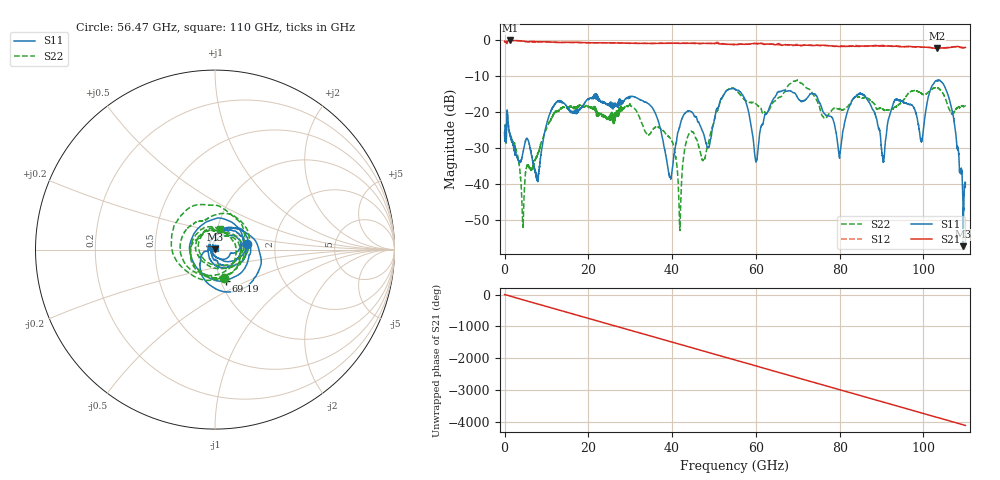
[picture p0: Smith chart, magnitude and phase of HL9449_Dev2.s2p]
! 5/9/2022 12:37:12 PM
! C:\USERS\VECTORSTARUSER\DESKTOP\JASON\HL9449-11\HL9449-11-NE04.S2P
! CHANNEL.1
! TR.MEASUREMENT
! CORRECTED.DATA
# GHZ S RI R 50.0
! FREQ.GHZ  S11RE  S11IM  S21RE  S21IM  S12RE  S12IM  S22RE  S22IM
!; PortSelection: Port_12
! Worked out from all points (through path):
!   5000 points, 22 MHz to 110 GHz, reference 50 ohm
!   highest |S21| = -0.24 dB at 1.386 GHz (marker M1); lowest = -2.4 dB at 103.2 GHz (marker M2)
!   group delay of S21, straight-line fit = 103 ps
!   lowest |S11| = -57.2 dB at 109.5 GHz (marker M3), VSWR 1.00, Z = 49.9 + j0.109 ohm
!   |S11| at or under -10 dB: start of sweep to end of sweep
!   |S22| runs from -52.9 to -11.3 dB; largest |S21 - S12| = 0.038
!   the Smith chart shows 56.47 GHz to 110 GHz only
!   S11 on the Smith chart (normalised r, x): 56.47 GHz: 1.44, +0.09; 69.19 GHz: 1.06, -0.38; 110 GHz: 1.00, +0.02
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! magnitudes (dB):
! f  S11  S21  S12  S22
! 22 MHz  -25.7  -0.5  -0.5  -25.6
! 1.386 GHz  -26.8  -0.2  -0.2  -26.9
! 4.4 GHz  -31.3  -0.4  -0.4  -51.4
! 18.37 GHz  -18.9  -0.8  -0.8  -18.4
! 36.7 GHz  -22.5  -1.1  -1.0  -24.3
! 39.51 GHz  -37.9  -1.0  -1.0  -27.3
! 41.84 GHz  -24.0  -1.1  -1.0  -52.2
! 44 GHz  -19.8  -1.0  -1.1  -26.2
! 48.58 GHz  -29.9  -1.1  -1.0  -29.0
! 55.02 GHz  -13.8  -1.3  -1.4  -13.7
! 56.47 GHz  -14.8  -1.3  -1.3  -15.5
! 60.06 GHz  -33.6  -1.1  -1.1  -17.8
! 69.19 GHz  -14.7  -1.6  -1.5  -11.5
! 73.35 GHz  -15.0  -1.6  -1.5  -14.6
! 79.93 GHz  -32.6  -1.9  -1.7  -19.4
! 84.46 GHz  -15.1  -1.9  -1.7  -15.8
! 91.67 GHz  -21.9  -1.8  -1.7  -19.4
! 99.55 GHz  -28.0  -2.1  -2.1  -15.0
! 103.2 GHz  -11.4  -2.4  -2.3  -13.4
! 109.5 GHz  -57.2  -2.2  -2.3  -18.5
! 110 GHz  -40.9  -2.2  -2.3  -18.5
! 110 GHz  -39.6  -2.2  -2.3  -18.5
